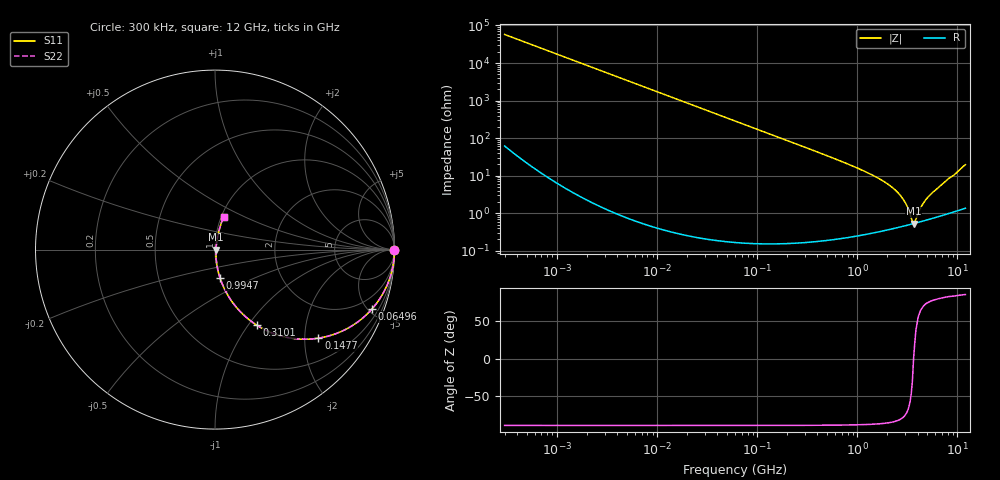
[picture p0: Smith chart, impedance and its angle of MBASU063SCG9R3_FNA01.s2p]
! MBASU063SCG9R3_FNA01  S-PARAMETER MODEL  ( General Type )
! Model Generated by TAIYO YUDEN Corporation (http://www.ty-top.com)
! Version 1.0
! TAIYO YUDEN Control No. 130801
! Copyright(c) 2013 TAIYO YUDEN CO.,LTD. All Rights Reserved.
! Product Description (link to TY-COMPAS)
! https://ds.yuden.co.jp/TYCOMPAS/or/detail?pn=MBASU063SCG9R3DFNA01&u=M
! Products Name : Multilayer Ceramic Capacitors
! Characteristics :
!  Capacitance : 9.3 pF , Rated Voltage : 50V , TCC : CG / C0G
!  Case Size : 0.6 x 0.3 / 0.024 x 0.012 [mm/inch] , Thickness : 0.3 / 0.012 [mm/inch]
!  (Conditions: Temperature = 25 degC , DC Bias Current/Voltage = 0A / 0V)
! External Node Assignments :
!  1  o---| |---o  2
! GND o---------o GND
! Frequency Range : 0.3MHz  -  12000MHz  [ 401 STEP ]
# MHz S RI R 50
! Freq[MHz].  S11 Real  S11 Imag  S21 Real  S21 Imag  S12 Real  S12 Imag  S22 Real  S22 Imag
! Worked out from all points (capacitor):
!   401 points, 300 kHz to 12 GHz, reference 50 ohm
!   read as one part in series: C = 9.23 pF near 316.3 kHz
!   lowest |Z| = 529 mohm at 3.643 GHz (marker M1)
!   series resonance near 3.646 GHz, so ESL is about 210 pH
!   S11 on the Smith chart (normalised r, x): 300 kHz: open; 64.96 MHz: 1.00, -5.31; 147.7 MHz: 1.00, -2.33; 310.1 MHz: 1.00, -1.10; 994.7 MHz: 1.00, -0.32; 12 GHz: 1.03, +0.39
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0.3  1 -0.00174  4.88e-06 0.00174  4.88e-06 0.00174  1 -0.00174
1.769972  0.9999 -0.0103  0.000108 0.0103  0.000108 0.0103  0.9999 -0.0103
10.44266  0.9963 -0.0603  0.00367 0.0603  0.00367 0.0603  0.9963 -0.0603
26.39317  0.9771 -0.1495  0.0229 0.1495  0.0229 0.1495  0.9771 -0.1495
60  0.8919 -0.3103  0.1081 0.3103  0.1081 0.3103  0.8919 -0.3103
64.96309  0.8755 -0.3298  0.1245 0.3298  0.1245 0.3298  0.8755 -0.3298
147.6816  0.5761 -0.4935  0.4239 0.4935  0.4239 0.4935  0.5761 -0.4935
310.0777  0.2344 -0.4221  0.7656 0.4221  0.7656 0.4221  0.2344 -0.4221
353.9943  0.1898 -0.3904  0.8102 0.3904  0.8102 0.3904  0.1898 -0.3904
555.3718  0.0858 -0.2769  0.9142 0.2769  0.9142 0.2769  0.0858 -0.2769
994.7115  0.0274 -0.1558  0.9726 0.1558  0.9726 0.1558  0.0274 -0.1558
2088.533  0.00673 -0.0551  0.9933 0.0551  0.9933 0.0551  0.00673 -0.0551
2514.07  0.00541 -0.0359  0.9946 0.0359  0.9946 0.0359  0.00541 -0.0359
2870.14  0.00501 -0.023  0.995 0.023  0.995 0.023  0.00501 -0.023
3107.553  0.00496 -0.0154  0.995 0.0154  0.995 0.0154  0.00496 -0.0154
3454.93  0.00511 -0.00542  0.9949 0.00542  0.9949 0.00542  0.00511 -0.00542
3642.919  0.00527 -5.46e-05  0.9947 5.46e-05  0.9947 5.46e-05  0.00527 -5.46e-05
3841.137  0.00548 0.00418  0.9945 -0.00418  0.9945 -0.00418  0.00548 0.00418
4502.883  0.00639 0.0162  0.9936 -0.0162  0.9936 -0.0162  0.00639 0.0162
5140.631  0.00747 0.0266  0.9925 -0.0266  0.9925 -0.0266  0.00747 0.0266
8966.534  0.0194 0.0938  0.9806 -0.0938  0.9806 -0.0938  0.0194 0.0938
12000  0.0491 0.1842  0.9509 -0.1842  0.9509 -0.1842  0.0491 0.1842
